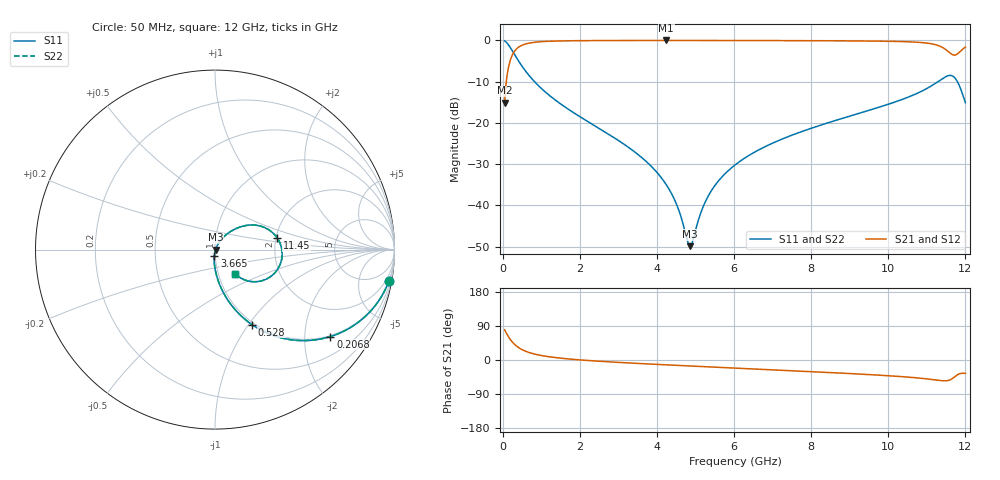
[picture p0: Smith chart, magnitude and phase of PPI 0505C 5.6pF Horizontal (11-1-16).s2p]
# MHz S MA R 50
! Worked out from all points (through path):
!   1601 points, 50 MHz to 12 GHz, reference 50 ohm
!   highest |S21| = -0.03 dB at 4.24 GHz (marker M1); lowest = -15.2 dB at 50 MHz (marker M2)
!   group delay of S21, straight-line fit = 17 ps
!   lowest |S11| = -49.9 dB at 4.86 GHz (marker M3), VSWR 1.01, Z = 50.3 - j0.0953 ohm
!   |S11| at or under -10 dB: 823.9 MHz to 11.29 GHz (10.47 GHz wide, 173 % of centre); 11.79 GHz to end of sweep
!   |S22| runs from -49.9 to -0.1 dB; largest |S21 - S12| = 0
!   S11 on the Smith chart (normalised r, x): 50 MHz: 1, -11; 206.8 MHz: 0.97, -2.68; 528 MHz: 0.97, -1.04; 3.665 GHz: 0.99, -0.07; 11.45 GHz: 2.04, +0.30; 12 GHz: 1.20, -0.33
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50  0.9846 -10.2  0.1748 79.8  0.1748 79.8  0.9846 -10.2
139.625  0.8956 -26.8  0.4442 63.1  0.4442 63.1  0.8956 -26.8
206.8438  0.8052 -37.0  0.592 52.9  0.592 52.9  0.8052 -37.0
356.2188  0.618 -52.9  0.7848 37.0  0.7848 37.0  0.618 -52.9
528  0.4666 -63.7  0.8828 26.1  0.8828 26.1  0.4666 -63.7
1013.469  0.2584 -78.0  0.9643 11.7  0.9643 11.7  0.2584 -78.0
2044.156  0.1155 -89.1  0.9912 -0.1  0.9912 -0.1  0.1155 -89.1
3664.875  0.03591 -95.7  0.9965 -9.9  0.9965 -9.9  0.03591 -95.7
4038.312  0.02389 -95.1  0.9967 -11.8  0.9967 -11.8  0.02389 -95.1
4239.969  0.01786 -93.5  0.9967 -12.8  0.9967 -12.8  0.01786 -93.5
4516.312  0.01008 -86.7  0.9966 -14.1  0.9966 -14.1  0.01008 -86.7
4859.875  0.003195 -17.2  0.9965 -15.8  0.9965 -15.8  0.003195 -17.2
5166.094  0.008799 50.4  0.9963 -17.2  0.9963 -17.2  0.008799 50.4
5352.812  0.01351 57.1  0.9961 -18.1  0.9961 -18.1  0.01351 57.1
6025  0.03081 61.6  0.9953 -21.3  0.9953 -21.3  0.03081 61.6
6839.094  0.05229 60.1  0.9938 -25.1  0.9938 -25.1  0.05229 60.1
8019.156  0.08641 55.7  0.9903 -30.7  0.9903 -30.7  0.08641 55.7
10013.31  0.1686 44.5  0.9737 -41.6  0.9737 -41.6  0.1686 44.5
11073.88  0.2726 29.6  0.9163 -50.7  0.9163 -50.7  0.2726 29.6
11447.31  0.3532 10.4  0.799 -54.9  0.799 -54.9  0.3532 10.4
11723.66  0.3517 -23.5  0.6625 -44.1  0.6625 -44.1  0.3517 -23.5
12000  0.1752 -49.9  0.8288 -35.3  0.8288 -35.3  0.1752 -49.9
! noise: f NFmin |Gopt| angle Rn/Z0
50  0.0008619  0.9385  0.8374  0.003126
1372  0.005019  0.7325  5.031  0.003735
2701  0.007878  0.676  9.167  0.004663
4031  0.01076  0.6524  13.27  0.005812
5360  0.01375  0.6425  17.33  0.007116
6682  0.01701  0.6424  21.32  0.008701
8012  0.02098  0.6533  25.3  0.01099
9341  0.02727  0.686  29.28  0.01582
1.067e+04  0.04825  0.7874  33.5  0.04289
1.2e+04  0.1507  0.9188  37.84  0.3669
